PROGRAM MAIN_CM

VAR CONSTANT
	// Configure spectrum analyzer here.
	cInitParsSpectrum	: ST_CM_MagnitudeSpectrum_InitPars :=(	nFFT_Length 		:= cFFTLength,                           
																nWindowLength		:= cWindowLength,
																nChannels			:= cMaxChannels,
																bTransformToDecibel	:= FALSE,
																eWindowType			:= cWindowType,
																nOverlap			:= cOverlap,								// edit value in GVL_Constants
																eScalingType		:= E_CM_ScalingType.eCM_RootPowerSum ); 
END_VAR
VAR		
	fbSpectrum						: FB_CMA_MagnitudeSpectrum := (stInitPars := cInitParsSpectrum, nOwnID := eID_Spectrum, aDestIDs := [eID_Sink]);
	
	bCalculateRecommendedOverlap	: BOOL := TRUE;
	nRecommendedOverlap				: UDINT;
	
	fbErrHist						: FB_HRErrHist; // error monitoring
	bGetChannelErrors				: BOOL := FALSE;
	aErrorList						: ARRAY[1..cMaxChannels] OF HRESULT;
	
	nChnIdx							: UDINT;
END_VAR

IF bCalculateRecommendedOverlap THEN
	nRecommendedOverlap := F_CM_CalculateRecommendedOverlap(eWindowType 		:= cWindowType,
															aWindowParameters 	:= cWindowParameters,
															nWindowLength 		:= cWindowLength);
	bCalculateRecommendedOverlap := FALSE;
END_IF

// Call Spectrum
fbSpectrum.Call();
IF fbSpectrum.bError THEN
	fbErrHist.AddError(bErr:=TRUE, hrErrCode:=fbSpectrum.hrErrorCode, sErrSource:='MAIN_CM.fbSpectrum'); // error monitoring
	IF fbSpectrum.hrErrorCode = E_CM_ErrorCode.eCM_ErrRTime_ErrornousChannelResults THEN
		bGetChannelErrors := fbSpectrum.GetChannelErrors(aErrorList);
		
		// ToDo: if channel error
	
	END_IF

	// ToDo: if general error
	
END_IF

// Get channel errors on info or error.
IF fbSpectrum.hrErrorCode = E_CM_ErrorCode.eCM_InfRTime_InvalidInputData OR fbSpectrum.hrErrorCode = E_CM_ErrorCode.eCM_InfRTime_AmbiguousChannelResults THEN
	bGetChannelErrors := fbSpectrum.GetChannelErrors(aErrorList);
	
	// ToDo: if channel info
	
END_IF

// ToDo: monitoring code

END_PROGRAM
